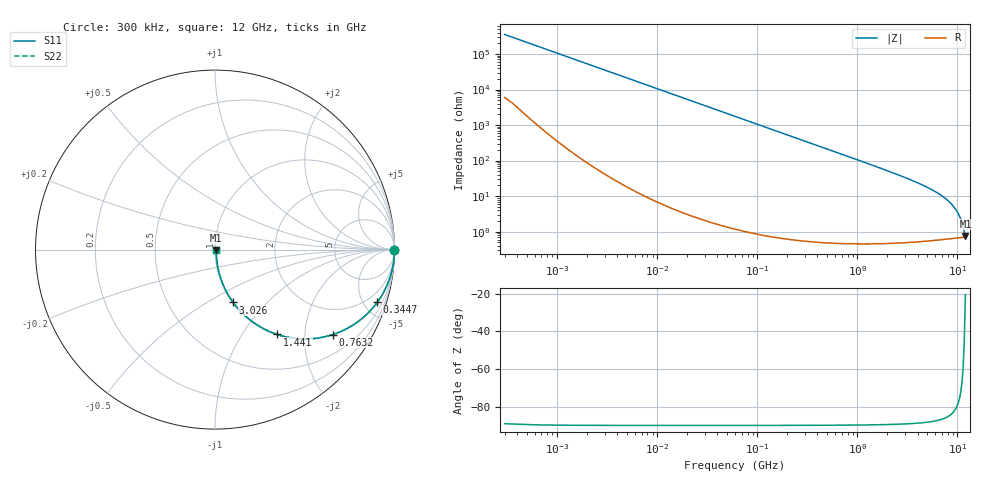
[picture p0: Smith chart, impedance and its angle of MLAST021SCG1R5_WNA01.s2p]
! MLAST021SCG1R5_WNA01  S-PARAMETER MODEL  ( General Type )
! Model Generated by TAIYO YUDEN Corporation (http://www.ty-top.com)
! Version 1.0
! TAIYO YUDEN Control No. 220901
! Copyright(c) 2022 TAIYO YUDEN CO.,LTD. All Rights Reserved.
! Product Description (link to TY-COMPAS)
! https://ds.yuden.co.jp/TYCOMPAS/or/detail?pn=MLAST021SCG1R5BWNA01&u=M
! Products Name : Multilayer Ceramic Capacitors
! Characteristics :
!  Capacitance : 1.5 pF , Rated Voltage : 25V , TCC : CG / C0G
!  Case Size : 0.25 x 0.125 / 0.0098 x 0.0049 [mm/inch] , Thickness : 0.125 / 0.0049 [mm/inch]
!  (Conditions: Temperature = 25 degC , DC Bias Current/Voltage = 0A / 0V)
! External Node Assignments :
!  1  o---| |---o  2
! GND o---------o GND
! Frequency Range : 0.3MHz  -  12000MHz  [ 401 STEP ]
# MHz S RI R 50
! Freq[MHz].  S11 Real  S11 Imag  S21 Real  S21 Imag  S12 Real  S12 Imag  S22 Real  S22 Imag
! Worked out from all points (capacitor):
!   401 points, 300 kHz to 12 GHz, reference 50 ohm
!   read as one part in series: C = 1.5 pF near 316.3 kHz
!   lowest |Z| = 751 mohm at 12 GHz (marker M1)
!   S11 on the Smith chart (normalised r, x): 300 kHz: open; 344.7 MHz: 1.01, -6.15; 763.2 MHz: 1.01, -2.77; 1.441 GHz: 1.01, -1.45; 3.026 GHz: 1.01, -0.66; 12 GHz: 1.01, -0.01
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0.3  1 -0.000283  4.84e-06 0.000283  4.84e-06 0.000283  1 -0.000283
1.769972  1 -0.00167  5.81e-06 0.00167  5.81e-06 0.00167  1 -0.00167
10.44266  0.9999 -0.00984  0.000103 0.00984  0.000103 0.00984  0.9999 -0.00984
60  0.9968 -0.0564  0.00322 0.0564  0.00322 0.0564  0.9968 -0.0564
151.6462  0.9798 -0.14  0.0202 0.14  0.0202 0.14  0.9798 -0.14
237.9135  0.9518 -0.2134  0.0482 0.2134  0.0482 0.2134  0.9518 -0.2134
344.7396  0.904 -0.2938  0.096 0.2938  0.096 0.2938  0.904 -0.2938
353.9943  0.8993 -0.3001  0.1007 0.3001  0.1007 0.3001  0.8993 -0.3001
526.7124  0.8011 -0.398  0.1989 0.398  0.1989 0.398  0.8011 -0.398
763.2128  0.6568 -0.4731  0.3432 0.4731  0.3432 0.4731  0.6568 -0.4731
1048.836  0.5021 -0.4978  0.4979 0.4978  0.4979 0.4978  0.5021 -0.4978
1441.349  0.346 -0.4726  0.654 0.4726  0.654 0.4726  0.346 -0.4726
2088.533  0.1979 -0.3937  0.8021 0.3937  0.8021 0.3937  0.1979 -0.3937
3026.31  0.1012 -0.2942  0.8988 0.2942  0.8988 0.2942  0.1012 -0.2942
5420.343  0.0292 -0.1516  0.9708 0.1516  0.9708 0.1516  0.0292 -0.1516
6699.894  0.0177 -0.1079  0.9823 0.1079  0.9823 0.1079  0.0177 -0.1079
8064.993  0.0115 -0.0726  0.9885 0.0726  0.9885 0.0726  0.0115 -0.0726
8966.534  0.00923 -0.0533  0.9908 0.0533  0.9908 0.0533  0.00923 -0.0533
9968.853  0.00779 -0.0346  0.9922 0.0346  0.9922 0.0346  0.00779 -0.0346
10793.46  0.00718 -0.0208  0.9928 0.0208  0.9928 0.0208  0.00718 -0.0208
11380.75  0.007 -0.0117  0.993 0.0117  0.993 0.0117  0.007 -0.0117
12000  0.00699 -0.00258  0.993 0.00258  0.993 0.00258  0.00699 -0.00258
